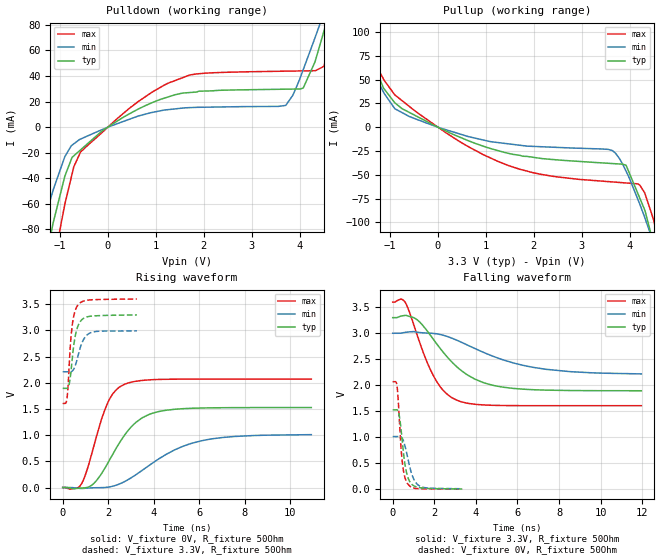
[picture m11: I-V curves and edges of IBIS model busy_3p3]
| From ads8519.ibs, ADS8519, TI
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|   busy_3p3 Model
[Model]   busy_3p3
Model_type   Output
Polarity   Non-Inverting
Vmeas = 1.65
Vref = 1.65
Cref = 5pF
Rref = 50
|   typ   min   max
|   (nom PVT)   (Fast PVT)   (slow PVT)
| C_comp by Frequency method (F=29Mhz)
|Average
|C_comp   6.278e-12   5.225e-12   7.515e-12
|ON state : BUFFER OUTPUT TURNED HIGH
|C_comp   6.278e-12   5.225e-12   7.515e-12
|OFF state: BUFFER OUTPUT TURNED LOW
|C_comp   6.893e-12   5.723e-12   7.748e-12
|C_comp by LC Tank method (L=1nH)
| Resonant frequency (Hz)  2.88e9   3.15e9   2.66e9
C_comp   3.057e-12   2.562e-12   3.584e-12
| Where nom  PVT is Nominal Process,  3.3V,  32C
|   Fast PVT is Strong Process,   3.6V,  -40C
|   Slow PVT is Weak Process,   3V,  92C
[Voltage Range]   3.3   3   3.6
|Ambient Temperature   25   85   -40
|Junction Temperature
[Temperature Range]   32   92   -40
[Pullup Reference]   3.3   3   3.6
[Pulldown Reference]   0   0   0
[Power Clamp Reference]   3.3   3   3.6
[GND Clamp Reference]   0   0   0
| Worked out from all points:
|   slope of the pulldown table from 0 to 0.495 V, typ, clamps not added: 43.5 ohm
|   slope of the pullup table from 0 to 0.495 V, typ, clamps not added: 43.7 ohm
|   falling waveform, V_fixture 3.3V, R_fixture 50Ohm: 20-80 % time 1.99ns typ, 3.16ns min, 1.25ns max; typ from 3.3 V to 1.89 V
|   rising waveform, V_fixture 0V, R_fixture 50Ohm: 20-80 % time 1.4ns typ, 2.35ns min, 894ps max; typ from 0 V to 1.53 V
|   rising waveform, V_fixture 3.3V, R_fixture 50Ohm: 20-80 % time 266ps typ, 349ps min, 210ps max; typ from 1.89 V to 3.3 V
|   falling waveform, V_fixture 0V, R_fixture 50Ohm: 20-80 % time 290ps typ, 391ps min, 221ps max; typ from 1.53 V to 0.005 V
[Pulldown]
|   Voltage   I(typ)   I(min)   I(max)
-3.3V     -567.5mA   -398.2mA   -790.3mA
-1.346V   -115.9mA   -77.42mA   -166.6mA
-1.134V   -74.07mA   -48.54mA   -106.8mA
-897.6mV  -38.47mA   -23.17mA   -60.53mA
-745.8mV  -23.66mA   -14.1mA    -36.72mA
-565.2mV  -17.68mA   -9.269mA   -19.34mA
1.246V    23.5mA     13.66mA    34.24mA
3.702V    29.71mA    16.98mA    43.82mA
4.072V    30.6mA     44.99mA    44.01mA
4.468V    70.43mA    85.77mA    46.91mA
5.023V    141.3mA    136.4mA    129.8mA
6.6V      258.6mA    235.3mA    294.2mA
[Pullup]
|   Voltage   I(typ)   I(min)   I(max)
-3.3V     226.9mA    203.5mA    263.7mA
-2.121V   151.6mA    130.4mA    179.8mA
-1.769V   117.3mA    97.07mA    139.1mA
-897mV    25.55mA    19.34mA    33.84mA
-285mV    7.331mA    5.216mA    10.11mA
1.465V    -27.48mA   -17.51mA   -40.17mA
3.636V    -38.21mA   -24.62mA   -57.51mA
3.924V    -40.08mA   -46.34mA   -58.61mA
4.212V    -74.88mA   -81.2mA    -60.96mA
4.468V    -117.2mA   -117.3mA   -92.96mA
4.655V    -158mA     -146.5mA   -136.1mA
6.6V      -610.4mA   -477.4mA   -756.6mA
[Ramp]
R_load = 50
|   typ   min   max
dV/dt_r   0.916652/1.39682e-09   0.607826/2.3592e-09   1.24242/8.9398e-10
dV/dt_f   0.843839/1.98322e-09   0.472967/3.21375e-09   1.19615/1.2445e-09
[Falling Waveform]
V_fixture = 3.3V
V_fixture_min = 3V
V_fixture_max = 3.6V
R_fixture = 50Ohm
|   Time   V(typ)   V(min)   V(max)
0s        3.3V       3V         3.6V
600ps     3.343V     3.017V     3.595V
1.18ns    3.258V     3.02V      2.961V
1.9ns     2.914V     2.998V     2.228V
2.42ns    2.64V      2.963V     1.906V
3.06ns    2.364V     2.87V      1.717V
3.98ns    2.113V     2.701V     1.633V
5.34ns    1.961V     2.484V     1.61V
7.4ns     1.906V     2.305V     1.607V
11.96ns   1.894V     2.218V     1.606V
[Rising Waveform]
V_fixture = 0V
V_fixture_min = 0V
V_fixture_max = 0V
R_fixture = 50Ohm
|   Time   V(typ)   V(min)   V(max)
0s        1.16nV     1.362nV    1.035nV
820ps     -9.237mV   -18.45mV   67.09mV
1.36ns    75.18mV    -4.832mV   779.2mV
2ns       480.7mV    8.028mV    1.639V
2.34ns    743.3mV    43.17mV    1.86V
2.72ns    1.003V     114.4mV    1.972V
3.22ns    1.245V     246.2mV    2.03V
3.94ns    1.418V     465.5mV    2.059V
6.08ns    1.518V     891.1mV    2.071V
10.92ns   1.528V     1.01V      2.071V
[Rising Waveform]
V_fixture = 3.3V
V_fixture_min = 3V
V_fixture_max = 3.6V
R_fixture = 50Ohm
|   Time   V(typ)   V(min)   V(max)
0s        1.894V     2.21V      1.606V
180ps     1.894V     2.21V      1.672V
220ps     1.902V     2.21V      1.844V
300ps     2.011V     2.209V     2.46V
400ps     2.376V     2.218V     3.028V
520ps     2.816V     2.294V     3.337V
660ps     3.073V     2.495V     3.48V
900ps     3.226V     2.813V     3.559V
1.2ns     3.271V     2.951V     3.582V
3.26ns    3.296V     2.992V     3.599V
[Falling Waveform]
V_fixture = 0V
V_fixture_min = 0V
V_fixture_max = 0V
R_fixture = 50Ohm
|   Time   V(typ)   V(min)   V(max)
0s        1.527V     1.014V     2.068V
200ps     1.527V     1.013V     2.005V
260ps     1.504V     1.014V     1.748V
320ps     1.408V     1.016V     1.334V
460ps     922.3mV    977.6mV    529mV
580ps     505.2mV    847.7mV    239.4mV
700ps     267.1mV    645.4mV    117.4mV
980ps     75.42mV    223.3mV    24.49mV
1.3ns     30.5mV     61.38mV    9.773mV
3.34ns    4.673mV    9.153mV    1.061mV
